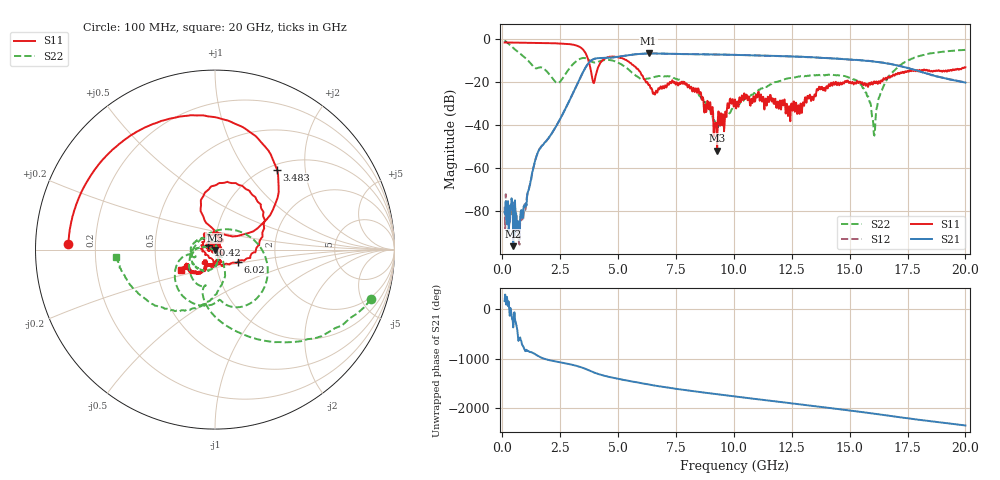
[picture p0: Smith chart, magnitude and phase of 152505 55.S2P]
!  2-Port S-parameters saved by WinCal
! VAR MeasName=S-Parameters (CALIBRATED_DATA) read from VNA (N5230C)
! VAR MeasDate=4/10/2015 9:34:14 AM
! VAR NAME=152505 55
! VAR FILENAME=152505 55.S2P
! VAR DATE=4/10/2015 9:34:14 AM
! VAR PHYS_PORTS=1,2
# Hz S DB R 50
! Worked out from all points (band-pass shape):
!   801 points, 100 MHz to 20 GHz, reference 50 ohm
!   highest |S21| = -6.80 dB at 6.319 GHz (marker M1); lowest = -96.2 dB at 473.1 MHz (marker M2)
!   |S21| within 3 dB of the highest: 3.877 GHz to 15.2 GHz (11.33 GHz wide, 119 % of centre)
!   lowest |S11| = -51.8 dB at 9.279 GHz (marker M3), VSWR 1.01, Z = 49.8 - j0.173 ohm
!   |S11| at or under -10 dB: 3.719 GHz to 4.331 GHz (611.7 MHz wide, 15.2 % of centre); 5.373 GHz to end of sweep
!   |S22| runs from -44.9 to -0.8 dB; largest |S21 - S12| = 0.0055
!   S11 on the Smith chart (normalised r, x): 100 MHz: 0.10, +0.02; 3.483 GHz: 1.09, +1.42; 6.02 GHz: 1.27, -0.18; 10.42 GHz: 0.93, +0.05; 20 GHz: 0.67, -0.16
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1e8  -1.75 177.6  -80.42 155.4  -77.92 94.2  -0.80 -17.7
4.73125e8  -1.77 168.8  -96.16 -12.3  -92.34 125.5  -4.26 -57.3
9.4575e8  -1.82 157.3  -77.31 -85.6  -78.61 -69.8  -8.44 -89.3
1.517875e9  -1.91 142.7  -53.23 142.3  -52.94 141.1  -13.61 -104.8
2.3885e9  -2.15 116.3  -39.37 16.1  -39.36 15.8  -20.54 124.7
3.43325e9  -4.47 57.5  -16.58 -97.4  -16.62 -97.2  -9.02 -44.1
3.483e9  -4.97 52.2  -15.54 -105.7  -15.55 -105.5  -8.92 -50.1
3.955625e9  -20.57 77.7  -9.38 163.3  -9.42 163.4  -10.99 -84.1
4.52775e9  -8.70 87.3  -8.83 82.0  -8.88 82.0  -9.82 -111.2
6.02025e9  -16.90 -28.6  -6.97 -56.1  -6.94 -56.0  -18.70 -164.0
6.31875e9  -21.51 -76.3  -6.80 -80.7  -6.83 -80.8  -18.40 -159.4
6.741625e9  -22.90 -172.9  -6.84 -113.2  -6.83 -113.5  -17.26 -167.4
8.458e9  -22.97 52.4  -7.22 133.4  -7.19 133.7  -25.31 106.8
9.278875e9  -51.84 -137.2  -7.32 84.7  -7.32 84.6  -39.72 29.4
1.005e10  -28.15 -179.7  -7.47 39.5  -7.49 39.4  -31.30 -51.9
1.042312e10  -26.87 146.1  -7.58 18.4  -7.56 18.4  -28.69 -65.7
1.199025e10  -28.61 101.3  -8.05 -70.1  -8.03 -69.9  -19.60 -95.1
1.338325e10  -26.85 -43.7  -8.62 -148.7  -8.59 -148.5  -16.90 -130.9
1.53235e10  -19.65 -131.8  -9.84 99.1  -9.82 98.4  -19.45 177.8
1.604488e10  -19.90 -125.6  -10.57 54.3  -10.53 53.8  -44.24 -126.3
1.669162e10  -17.49 -115.4  -11.57 13.1  -11.56 12.4  -17.36 -65.8
2e10  -13.25 -149.2  -20.33 177.1  -20.32 177.6  -5.12 -175.9
